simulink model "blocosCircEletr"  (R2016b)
settings: Solver=ode45  StartTime=0.0  StopTime=600*5  FixedStep=1  RelTol=1e-6  EnableMultiTasking=on
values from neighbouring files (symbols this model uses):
  C2 = zpk(-1/ans,[],1)    [PID_Sevilla.m]
undefined symbols (not defined in the file or in its folder): C4, L3, L5, R1, R6

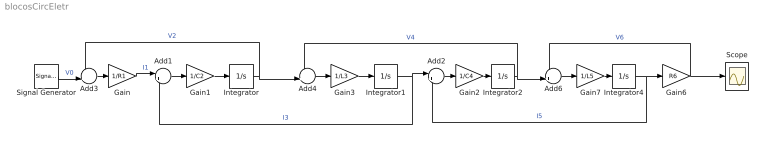
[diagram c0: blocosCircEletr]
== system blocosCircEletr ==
  Add1 : Sum  Inputs=|+-
  Add2 : Sum  Inputs=|+-
  Add3 : Sum  Inputs=-+|
  Add4 : Sum  Inputs=-+|
  Add6 : Sum  Inputs=-+|
  Gain : Gain  Gain=1/R1
  Gain1 : Gain  Gain=1/C2
  Gain2 : Gain  Gain=1/C4
  Gain3 : Gain  Gain=1/L3
  Gain6 : Gain  Gain=R6
  Gain7 : Gain  Gain=1/L5
  Integrator{,1..2,4} (4 alike) : Integrator
  Scope : Scope
  Signal Generator : SignalGenerator  WaveForm=square  Amplitude=20  Frequency=1/500
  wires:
  Signal Generator/1 -> Add3/2  "V0"
  Gain1/1 -> Integrator/1
  Add3/1 -> Gain/1
  Add1/1 -> Gain1/1
  Gain/1 -> Add1/1  "I1"
  Integrator/1 -> Add4/2, Add3/1  "V2"
  Gain3/1 -> Integrator1/1
  Add4/1 -> Gain3/1
  Gain2/1 -> Integrator2/1
  Integrator1/1 -> Add1/2, Add2/1  "I3"
  Integrator2/1 -> Add6/2, Add4/1  "V4"
  Gain7/1 -> Integrator4/1
  Add6/1 -> Gain7/1
  Integrator4/1 -> Add2/2, Gain6/1  "I5"
  Gain6/1 -> Scope/1, Add6/1  "V6"
  Add2/1 -> Gain2/1
